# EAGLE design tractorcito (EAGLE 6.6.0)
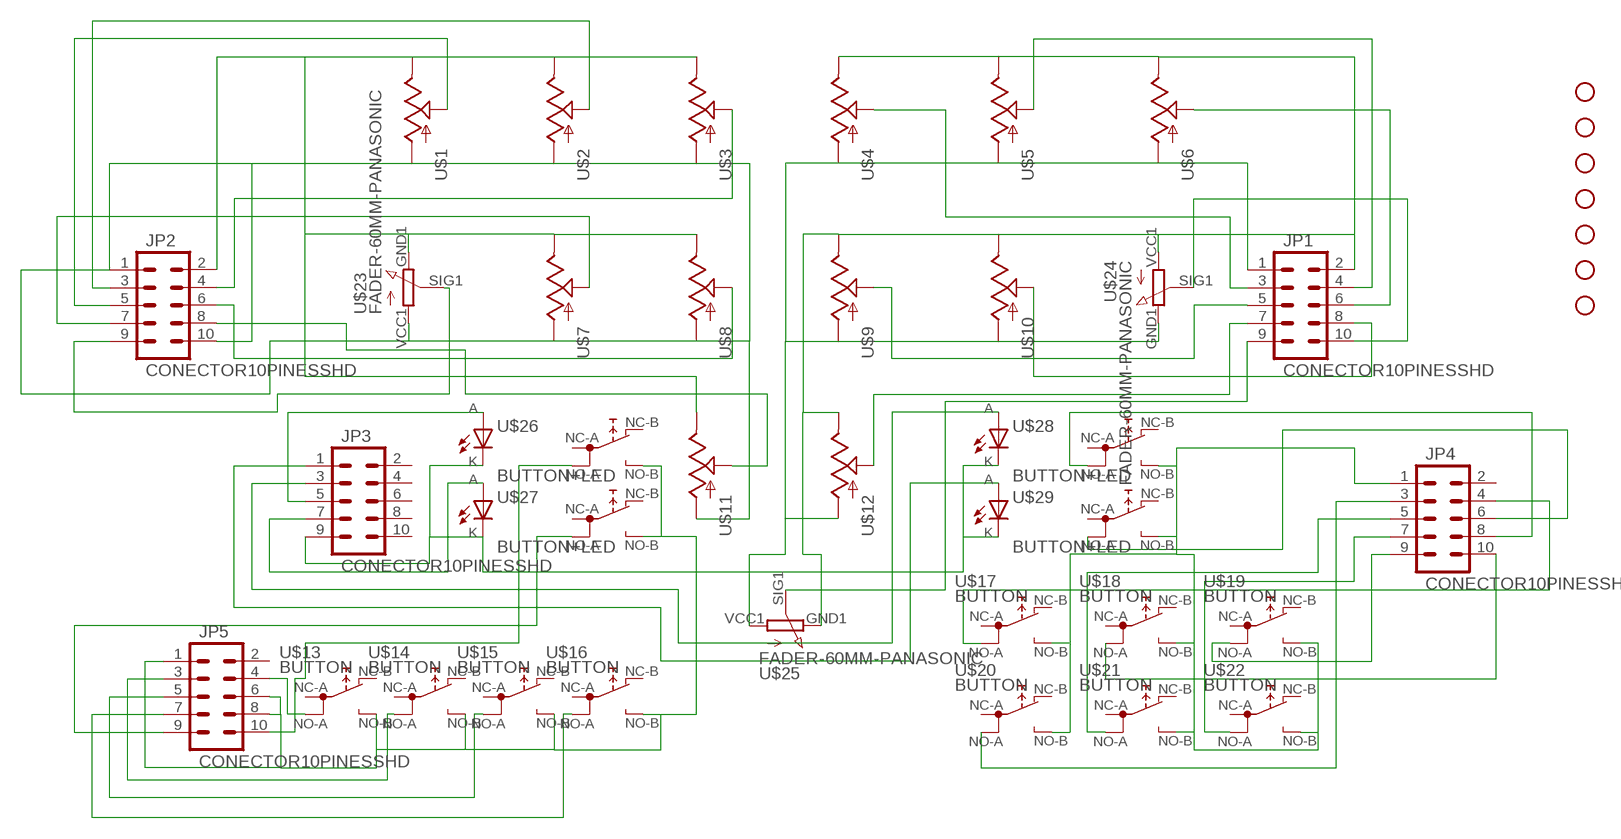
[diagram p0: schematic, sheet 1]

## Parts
JP1  CONECTOR10PINESSHD  [CONECTOR10PINES]
JP2  CONECTOR10PINESSHD  [CONECTOR10PINES]
JP3  CONECTOR10PINESSHD  [CONECTOR10PINES]
JP4  CONECTOR10PINESSHD  [CONECTOR10PINES]
JP5  CONECTOR10PINESSHD  [CONECTOR10PINES]
STANDOFF1  STAND-OFF  [STAND-OFF]
STANDOFF2  STAND-OFF  [STAND-OFF]
STANDOFF3  STAND-OFF  [STAND-OFF]
STANDOFF4  STAND-OFF  [STAND-OFF]
STANDOFF5  STAND-OFF  [STAND-OFF]
STANDOFF6  STAND-OFF  [STAND-OFF]
STANDOFF7  STAND-OFF  [STAND-OFF]
U$1  POT  [ALPS_POT]
U$2  POT  [ALPS_POT]
U$3  POT  [ALPS_POT]
U$4  POT  [ALPS_POT]
U$5  POT  [ALPS_POT]
U$6  POT  [ALPS_POT]
U$7  POT  [ALPS_POT]
U$8  POT  [ALPS_POT]
U$9  POT  [ALPS_POT]
U$10  POT  [ALPS_POT]
U$11  POT  [ALPS_POT]
U$12  POT  [ALPS_POT]
U$13  BUTTON  [BUTTON]
U$14  BUTTON  [BUTTON]
U$15  BUTTON  [BUTTON]
U$16  BUTTON  [BUTTON]
U$17  BUTTON  [BUTTON]
U$18  BUTTON  [BUTTON]
U$19  BUTTON  [BUTTON]
U$20  BUTTON  [BUTTON]
U$21  BUTTON  [BUTTON]
U$22  BUTTON  [BUTTON]
U$23  FADER-60MM-PANASONIC  [FADER-60MM-PANASONIC]
U$24  FADER-60MM-PANASONIC  [FADER-60MM-PANASONIC]
U$25  FADER-60MM-PANASONIC  [FADER-60MM-PANASONIC]
U$26  BUTTON+LED  [BUT+LED]
U$27  BUTTON+LED  [BUT+LED]
U$28  BUTTON+LED  [BUT+LED]
U$29  BUTTON+LED  [BUT+LED]

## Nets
N$1: JP2.2 U$1.P$1(E) U$2.P$1(E) U$3.P$1(E) U$7.P$1(E) U$8.P$1(E) U$11.P$1(E) U$23.GND1
N$2: JP3.9 U$26.K(C) U$27.K(C) U$28.K(C) U$29.K(C)
N$3: JP2.3 U$2.P$2(S)
N$4: JP2.5 U$1.P$2(S)
N$5: JP1.10 U$24.SIG1
N$6: JP2.7 U$7.P$2(S)
N$7: JP2.4 U$3.P$2(S)
N$8: JP2.6 U$8.P$2(S)
N$10: JP1.2 U$4.P$1(E) U$5.P$1(E) U$6.P$1(E) U$9.P$1(E) U$10.P$1(E) U$12.P$1(E) U$24.VCC1 U$25.GND1
N$11: JP1.4 U$5.P$2(S)
N$12: JP1.1 U$4.P$3(A) U$5.P$3(A) U$6.P$3(A) U$9.P$3(A) U$10.P$3(A) U$12.P$3(A) U$24.GND1 U$25.VCC1
N$13: JP1.6 U$6.P$2(S)
N$15: JP1.8 U$10.P$2(S)
N$16: JP1.3 U$4.P$2(S)
N$17: JP1.5 U$9.P$2(S)
N$18: JP1.7 U$12.P$2(S)
N$19: JP4.10 U$18.P$5(1B)
N$20: JP1.9 U$25.SIG1
N$21: JP3.5 U$26.A
N$22: JP3.7 U$27.A
N$23: JP2.9 U$23.SIG1
N$24: JP3.3 U$28.A
N$25: JP3.1 U$29.A
N$26: JP2.1 JP2.10 U$1.P$3(A) U$2.P$3(A) U$3.P$3(A) U$7.P$3(A) U$8.P$3(A) U$11.P$3(A) U$23.VCC1
N$27: JP5.4 U$13.P$5(1B)
N$28: JP5.3 U$14.P$5(1B)
N$29: JP5.5 U$15.P$5(1B)
N$30: JP5.7 U$16.P$5(1B)
N$31: JP5.9 U$27.P$5(1B)
N$32: JP5.10 U$26.P$5(1B)
N$33: JP4.1 U$17.P$6(NO) U$18.P$6(NO) U$19.P$6(NO) U$20.P$6(NO) U$21.P$6(NO) U$22.P$6(NO) U$28.P$6(NO) U$29.P$6(NO)
N$34: JP4.9 U$19.P$5(1B)
N$35: JP4.7 U$22.P$5(1B)
N$36: JP4.5 U$21.P$5(1B)
N$37: JP4.3 U$20.P$5(1B)
N$38: JP4.8 U$28.P$5(1B)
N$39: JP4.4 U$17.P$5(1B)
N$40: JP4.6 U$29.P$5(1B)
N$41: JP5.1 JP5.6 JP5.8 U$13.P$6(NO) U$14.P$6(NO) U$15.P$6(NO) U$16.P$6(NO) U$26.P$6(NO) U$27.P$6(NO)
N$42: JP2.8 U$11.P$2(S)
Unconnected: JP3.2 JP3.4 JP3.6 JP3.8 JP3.10 JP4.2 JP5.2 U$13.P$1(1A) U$13.P$2(NC) U$14.P$1(1A) U$14.P$2(NC) U$15.P$1(1A) U$15.P$2(NC) U$16.P$1(1A) U$16.P$2(NC) U$17.P$1(1A) U$17.P$2(NC) U$18.P$1(1A) U$18.P$2(NC) U$19.P$1(1A) U$19.P$2(NC) U$20.P$1(1A) U$20.P$2(NC) U$21.P$1(1A) U$21.P$2(NC) U$22.P$1(1A) U$22.P$2(NC) U$26.P$1(1A) U$26.P$2(NC) U$27.P$1(1A) U$27.P$2(NC) U$28.P$1(1A) U$28.P$2(NC) U$29.P$1(1A) U$29.P$2(NC)

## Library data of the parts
JP1-JP5 = tcmidi:CONECTOR10PINES: Header 5x2 Standard 10-pin dual row 0.1" header. Commonly used with AVR-ISP. Use with Spark Fun Electronics SKU: PRT-00778
STANDOFF1-STANDOFF7 = SparkFun-Electromechanical:STAND-OFF: #4 Stand Off
U$1-U$12 = SparkFun-Electromechanical:POT
U$13-U$22 = tcmidi:BUTTON
U$23-U$25 = tcmidi:FADER-60MM-PANASONIC
U$26-U$29 = tcmidi:BUTTON+LED

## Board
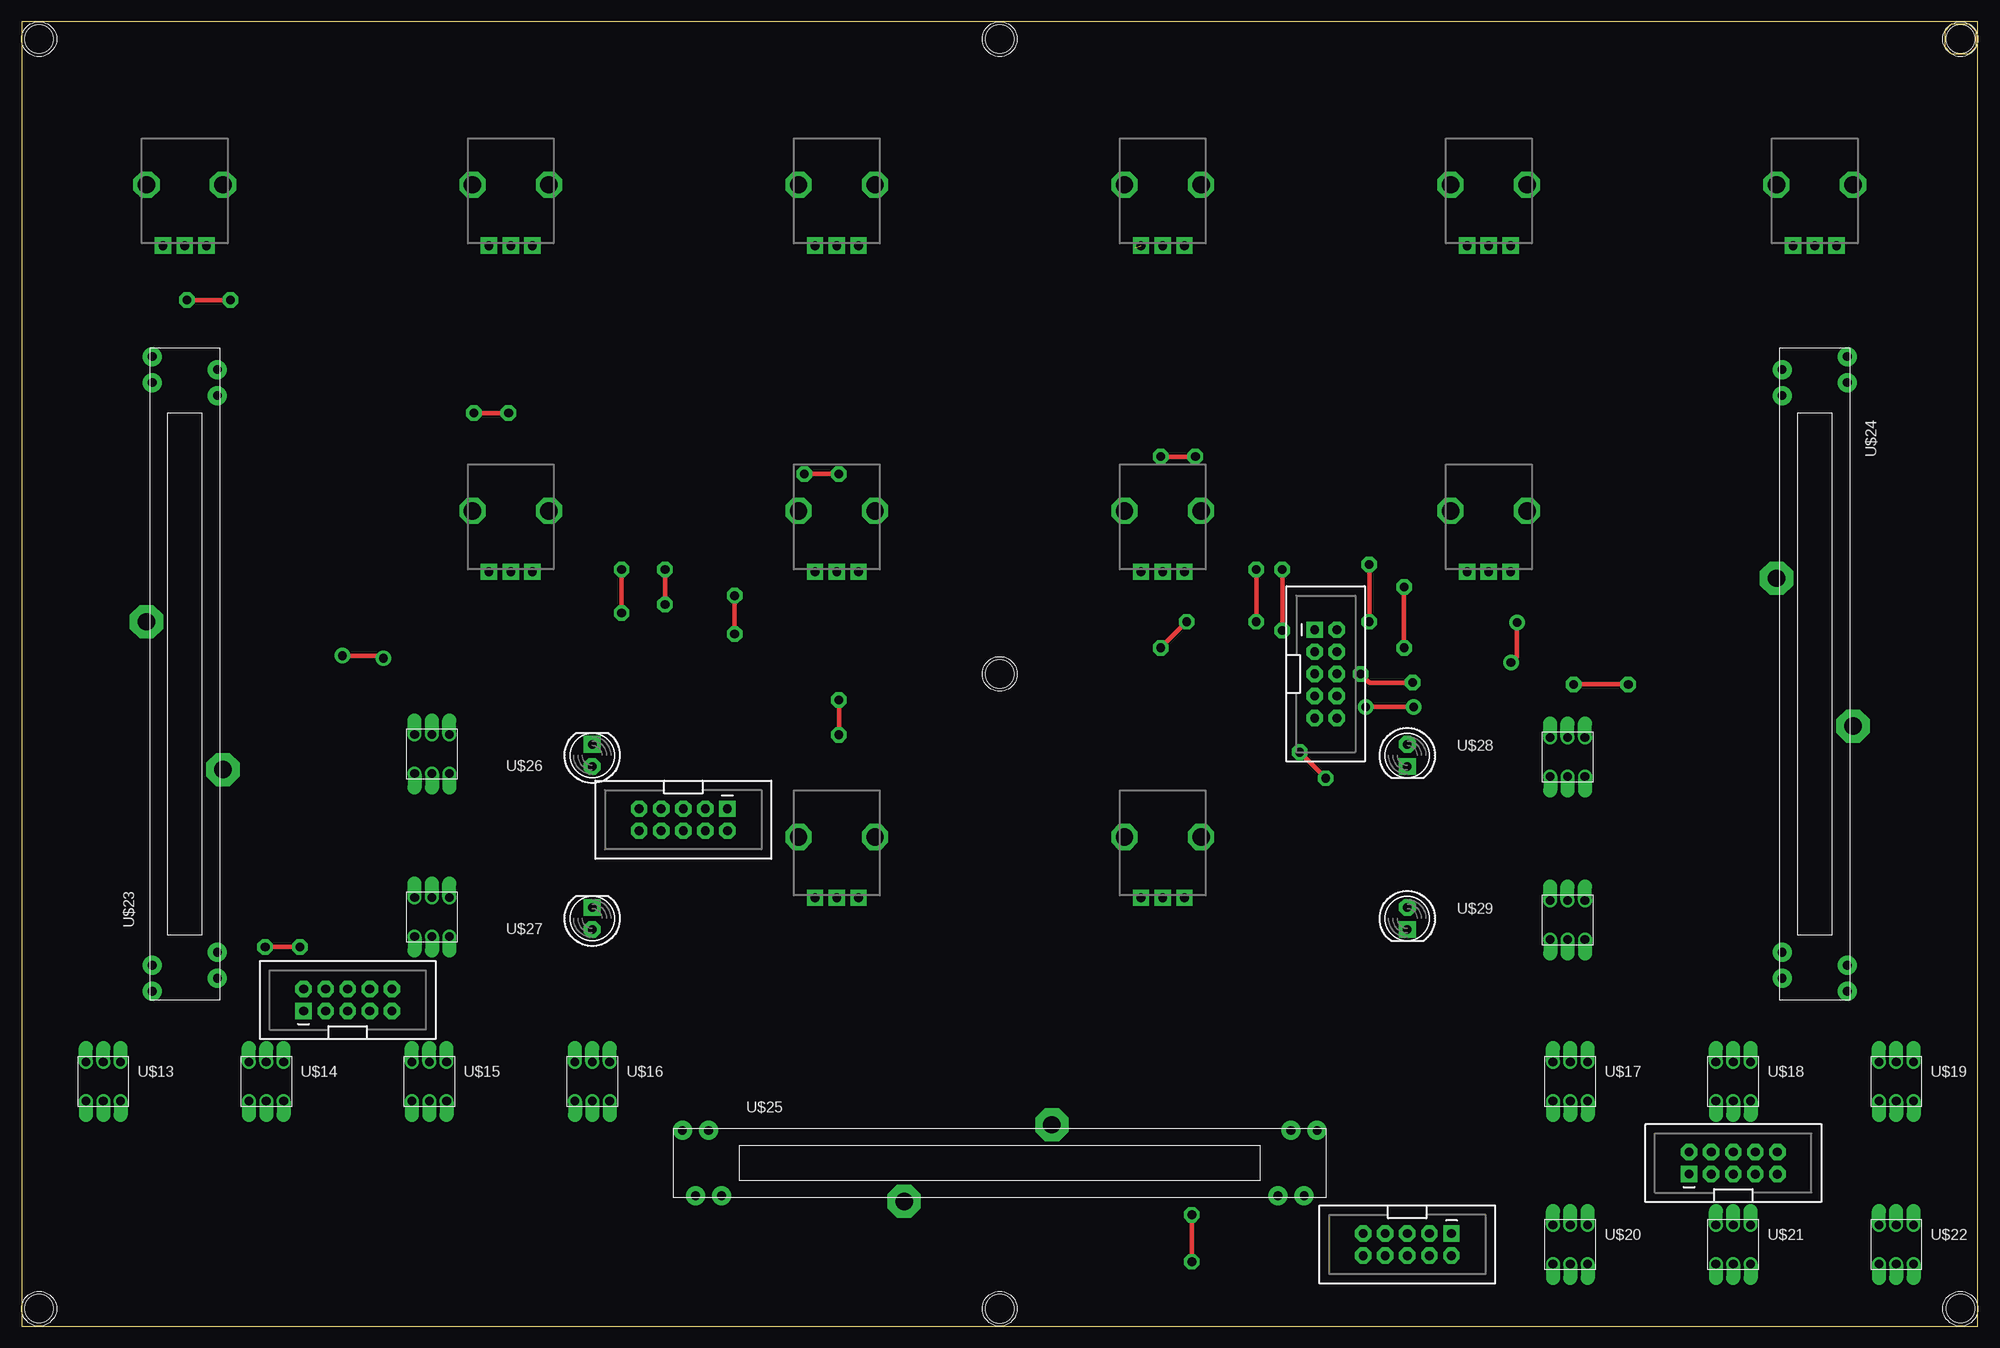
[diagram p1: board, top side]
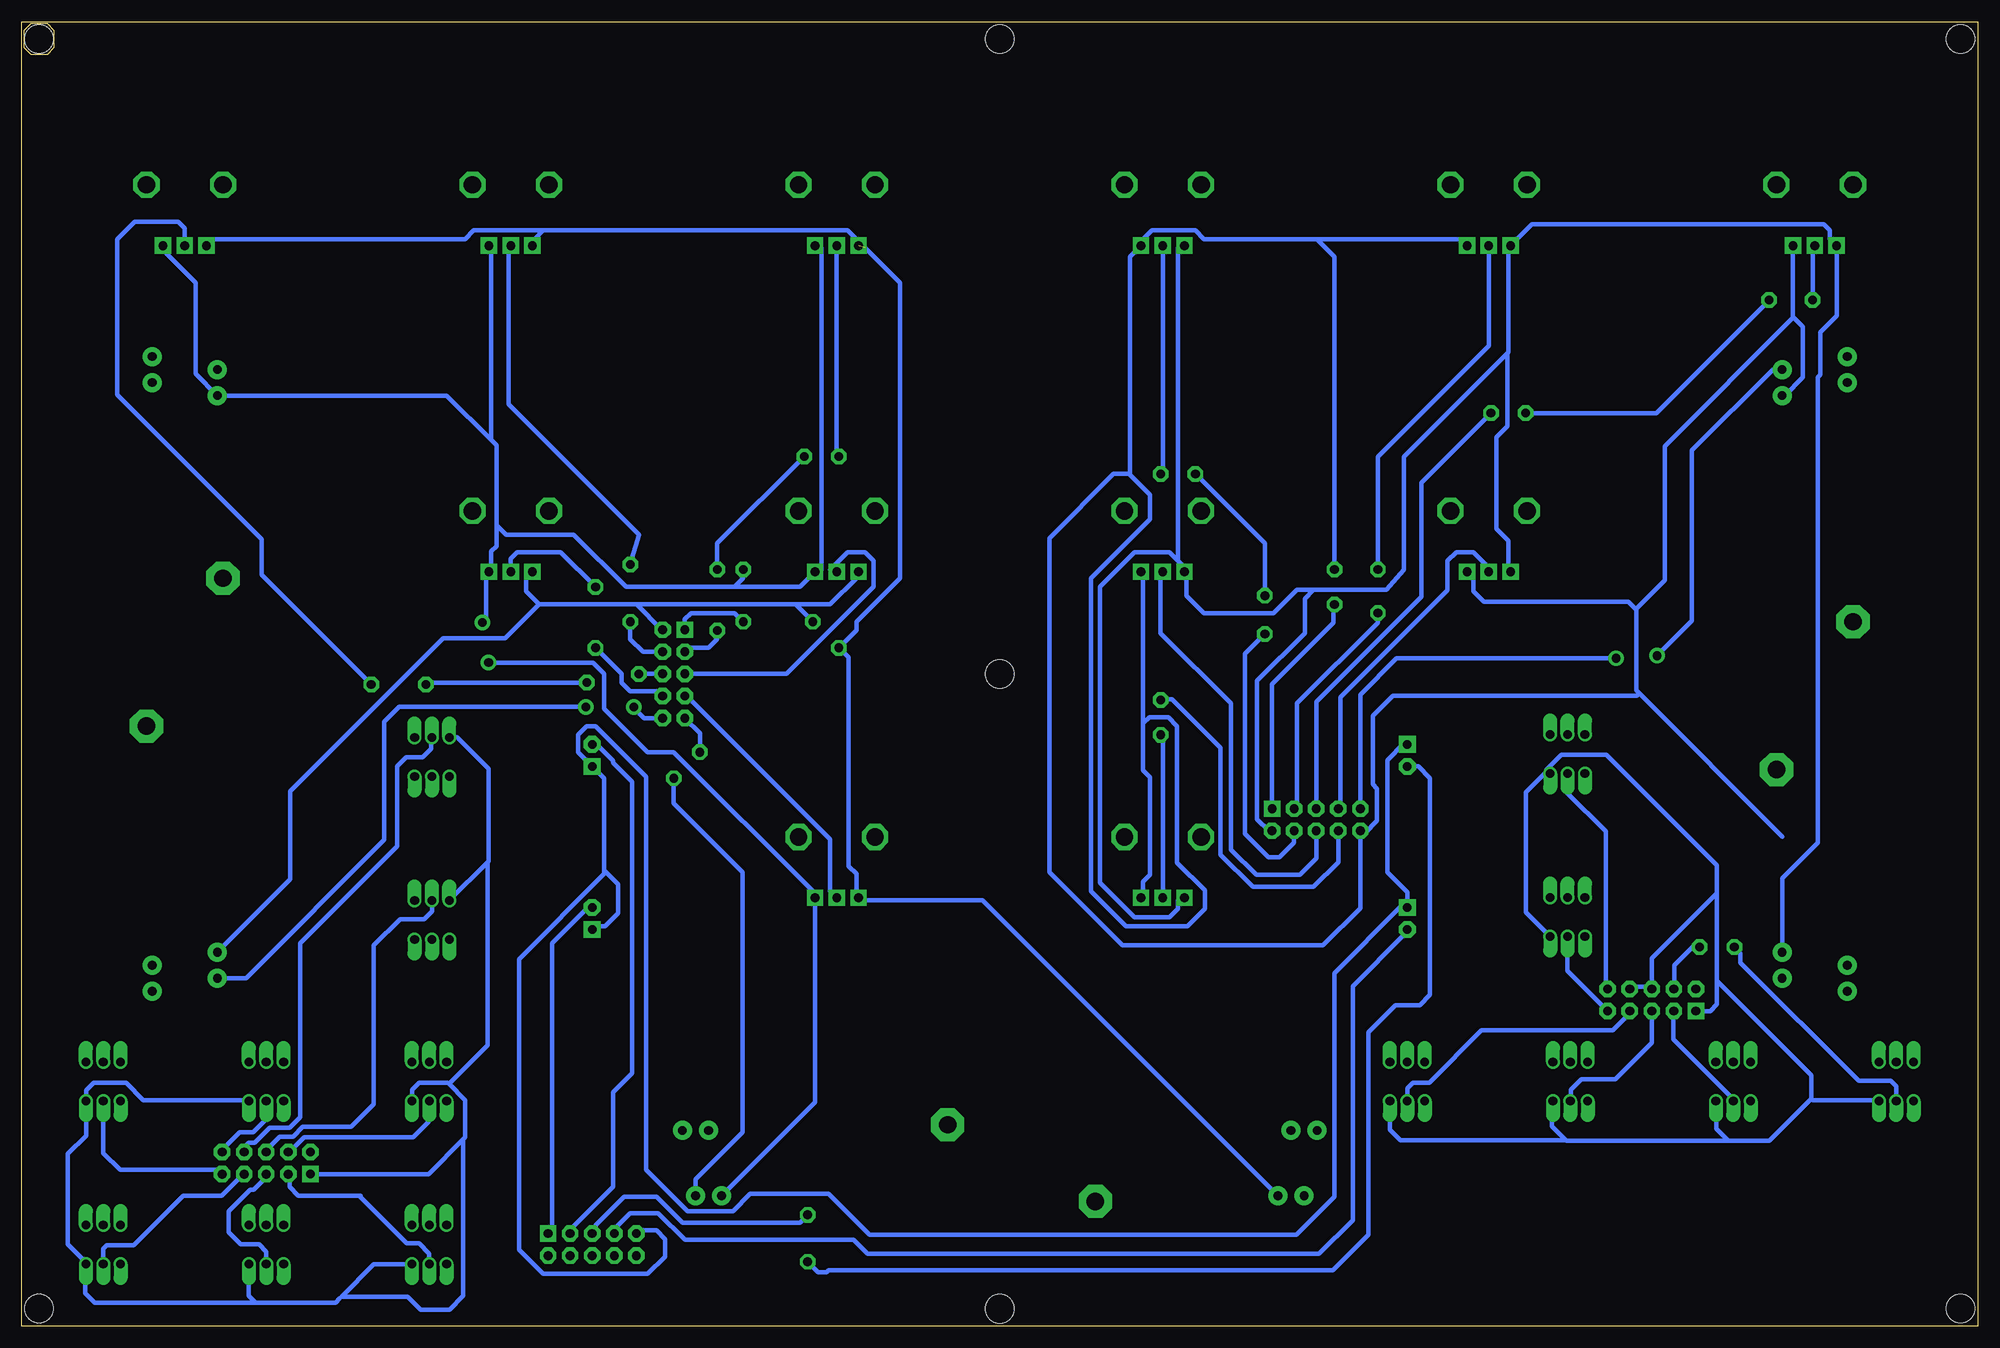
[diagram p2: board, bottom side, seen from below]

Size 225 x 150 mm. Coordinates in mm from the lower left corner, seen from the top.
Outline: 0,0 225,0 225,150 0,150 0,0
Outline: 224.75,147.04 223.97,146.26 222.04,146.26 221.25,147.04 221.25,148.97 222.04,149.76 223.97,149.76 224.75,148.97 224.75,147.04
Copper layers (1*16): Top 0.035mm / dielectric 1.5mm / Bottom 0.035mm
Design rules "tcmidi *": minimum track width 14mil, minimum drill 20mil, track to track 16mil, track to pad 16mil, pad to pad 12mil, via to via 16mil, smd to smd 16mil, copper to edge 16mil, drill to drill 16mil, minimum pad ring 12mil, minimum via ring 10mil, stop-mask expansion 4mil, vias tented up to drill 20mil, thermal gap 10mil

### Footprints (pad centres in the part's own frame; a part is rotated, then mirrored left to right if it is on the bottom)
CONECTOR10PINES = drill 1 pad 1.88 square: 1 -1.27,5.08 | drill 1.016 pad 1.88 octagon: 2 1.27,5.08; 3 -1.27,2.54; 4 1.27,2.54; 5 -1.27,0; 6 1.27,0; 7 -1.27,-2.54; 8 1.27,-2.54; 9 -1.27,-5.08; 10 1.27,-5.08
STAND-OFF = hole 3.302: 0,0
ALPS_POT = drill 1 pad 1.88 square: P$1 7,-2.5; P$2 7,0; P$3 7,2.5 | drill 2 octagon: P$4 0,-4.4; P$5 0,4.4
BUTTON = drill 1 pad 1.5 offset: P$1 -2,2.25; P$2 0,2.25; P$3 2,2.25; P$4 -2,-2.25; P$5 0,-2.25; P$6 2,-2.25
FADER-60MM-PANASONIC = drill 1 pad 2.184: GND1 -32,-3.75; GND2 -33.5,3.75; GND11 -35,-3.75; GND22 -36.5,3.75; SIG1 35,-3.75; SIG2 36.5,3.75; VCC1 32,-3.75; VCC2 33.5,3.75 | drill 2 pad 3.81 octagon: P$9 -11,-4.4; P$10 6,4.4
BUT+LED = drill 1 pad 1.93 octagon: A -9.375,1.27 | drill 1 pad 1.93 square: K -9.375,-1.27 | drill 1 pad 1.5 offset: P$1 11.06,-2.42; P$2 9.06,-2.42; P$3 7.06,-2.42; P$4 11.06,2.08; P$5 9.06,2.08; P$6 7.06,2.08

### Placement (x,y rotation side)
JP1  150,75 0 top
JP2  76.1,58.23 270 top
JP3  159.38,9.38 270 top
JP4  196.88,18.75 90 top
JP5  37.5,37.5 90 top
STANDOFF1  2,2 0 top
STANDOFF2  112.5,1.99 0 top
STANDOFF3  223,2 0 top
STANDOFF4  2,148 0 top
STANDOFF5  112.5,148 0 top
STANDOFF6  223,148 0 top
STANDOFF7  112.5,75 0 top
U$1  18.75,131.25 270 top
U$2  56.25,131.25 270 top
U$3  93.75,131.25 270 top
U$4  131.25,131.25 270 top
U$5  168.75,131.25 270 top
U$6  206.25,131.25 270 top
U$7  56.25,93.75 270 top
U$8  93.75,93.75 270 top
U$9  131.25,93.75 270 top
U$10  168.75,93.75 270 top
U$11  93.75,56.25 270 top
U$12  131.25,56.25 270 top
U$13  9.38,28.12 0 top
U$14  28.12,28.12 0 top
U$15  46.88,28.12 0 top
U$16  65.62,28.12 0 top
U$17  178.12,28.12 0 top
U$18  196.88,28.12 0 top
U$19  215.62,28.12 0 top
U$20  178.12,9.38 0 top
U$21  196.88,9.38 0 top
U$22  215.62,9.38 0 top
U$23  18.75,75 90 top
U$24  206.25,75 270 top
U$25  112.5,18.75 0 top
U$26  56.25,65.62 180 top
U$27  56.25,46.88 180 top
U$28  168.75,65.62 0 top
U$29  168.75,46.88 0 top

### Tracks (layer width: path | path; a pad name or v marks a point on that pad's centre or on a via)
N$1
  Bottom 0.508: U$7.P$1 54,87 54,90.3 55.4,91.7 55.4,102.2 54.1,103.5 54.1,111.9 | 92,88 91,87 U$8.P$1 91,86 91,84 89,82 81.03,82 78.34,84.65 76.4,84.66 | 92,88 93,89 97,89 101,85 101,51 97,47 93,47 92,48 92,49 U$11.P$1 | 92,88 92,124 U$3.P$1 | 54.1,111.9 66,100 66,87 68.03,84.68 76.4,84.66 | 54.1,111.9 54,112 54,124 U$2.P$1 51.3,126.7 17.7,126.7 17,126 17,125 U$1.P$1 16.2,124.2 16.2,116.2 18.1,114.3 18.1,109.4 18.4,109.1 18.4,55.6 22.5,51.5 U$23.GND1 | JP2.2 81.56,56.95 82.9,58.3 82.9,74.2 77.4,79.7 77.4,83.66 76.4,84.66
N$2
  Bottom 0.508: U$26.K 66,67 67.9,65.1 67.9,52.2 65.6,49.9 65.6,48.17 U$27.K 66.45,48.15 74,40.6 74,14.9 78.4,10.5 127.5,10.5 132.2,15.2 141.2,15.2 143.2,13.2 148.4,13.2 153.2,18 153.2,63.2 159,69 160,69 161,68 161,66 160,65 U$28.K 159,64 158,63 158,52.4 | 158,52.4 158,52 167.8,42.2 167.8,8.8 165,6 153,6 151,8 151,10 152,11 153.94,11 JP3.9 | U$29.K 159,46 157.9,46 156.4,47.5 156.4,50.8 158,52.4
N$3  (via drill 1 pad 1.78)
  Top 0.508: v69,87 v69,82
  Bottom 0.508: U$2.P$2 56.25,112.75 69,100 v69,87 | v69,82 69,80.9 78.3,71.6 78.3,59.84 JP2.3
N$4  (via drill 1 pad 1.78)
  Top 0.508: v56,105 v52,105 | v24,118 v19,118
  Bottom 0.508: v56,105 64,97 64,83.9 76.1,71.8 JP2.5 | v52,105 37,105 v24,118 | v19,118 19,124 U$1.P$2
N$5  (via drill 1 pad 1.78)
  Top 0.508: v160.1,71.2 v154.6,71.2
  Bottom 0.508: U$24.SIG1 199.2,40 183.3,55.9 183.3,69.5 181.6,71.2 v160.1,71.2 | v154.6,71.2 154.6,71.1 153.4,69.9 151.29,69.9 JP1.10
N$6
  Bottom 0.508: U$7.P$2 56,87 58,89 60,89 61,88 61,84.6 73.3,72.3 73.3,59.76 JP2.7
N$7  (via drill 1 pad 1.78)
  Top 0.508: v94,98 v90,98 | v82,84 v82,79.6
  Bottom 0.508: U$3.P$2 93.75,98.25 v94,98 | v82,84 82,90 v90,98 | JP2.4 78.64,55.56 80.3,53.9 81.6,53.9 84.3,56.6 84.3,77.3 v82,79.6
N$8
  Bottom 0.508: JP2.6 76.1,53.8 78,51.9 83,51.9 85.9,54.8 85.9,71.6 94,79.7 94,86.5 U$8.P$2
N$10  (via drill 1 pad 1.78)  (1 unrouted)
  Top 0.508: v131,78 v134,81
  Bottom 0.508: U$10.P$1 167,86 167,84.5 165.5,83 | 154.3,83 136,83 | U$9.P$1 129,86 132,83 136,83 | 128,124 124,120 124,86 129,81 129,80 v131,78 129.9,76.9 129.9,52.9 129,52 129,50 U$12.P$1 128,49 114.5,49 U$25.GND1 | v134,81 136,83 | 165,126 130,126 129,125 U$4.P$1 | 165,126 166,125 U$5.P$1 | 165,126 173,126 174,125 203,125 U$6.P$1 | JP1.2 151.38,80.08 154.3,83 | 165.5,83 154.3,83 | 165.5,83 169.4,79.1 176.5,79.1 194.1,61.5 194.1,51.4 U$24.VCC1
N$11  (via drill 1 pad 1.78)
  Top 0.508: v155,81 v155,87.6
  Bottom 0.508: JP1.4 153.54,77.54 155,79 v155,81 | v155,87.6 154,91 169,106 169,124 U$5.P$2
N$12  (via drill 1 pad 1.78)
  Top 0.508: v142,81 v142,87 | v172,80.9 172,77 v171.3,76.3
  Bottom 0.508: U$4.P$3 133,124 133,87 U$9.P$3 135.5,85 143,85 | U$6.P$3 209,124 205,120 205,109.5 U$24.GND1 176.1,107 171,101.9 | 171,101.9 171,124 U$5.P$3 | 143,85 155.5,85 161.5,91 169.3,91 170.4,92.1 | JP1.1 148.73,81.27 148,82 143,82 v142,81 | v142,87 142,86 143,85 | 170.4,92.1 170.4,89.7 171,89.1 171,87 U$10.P$3 171.6,86.4 171.6,81.3 v172,80.9 | 170.4,92.1 170.4,101.3 171,101.9 | U$25.VCC1 133.75,25.75 U$12.P$3 134,50 150,66 153,66 158,71 158,75 159.3,76.3 v171.3,76.3
N$13  (via drill 1 pad 1.78)
  Top 0.508: v184.8,73.8 v178.5,73.8 | v160,74 155,74 v154,75
  Bottom 0.508: U$6.P$2 206.25,126.25 207,127 212,127 214,125 214,107.1 197.4,90.5 197.4,86.4 v184.8,73.8 | v178.5,73.8 178,74 v160,74 | v154,75 JP1.6
N$15  (via drill 1 pad 1.78)
  Top 0.508: v159,85 v159,78
  Bottom 0.508: U$10.P$2 168.75,88.25 168,89 163,89 v159,85 | v159,78 156,75 156,74 155,73 151.81,73 JP1.8
N$16  (via drill 1 pad 1.78)
  Top 0.508: v131,100 v135,100 | v145,87 v145,80
  Bottom 0.508: U$4.P$2 131.25,100.25 v131,100 | v135,100 145,90 v145,87 | v145,80 145,79 146,78 148.27,78 JP1.3
N$17
  Bottom 0.508: JP1.5 137,75 127,85 127,88 128,89 130,89 132,87 U$9.P$2
N$18
  Bottom 0.508: U$12.P$2 132,50 132,56 148,72 JP1.7
N$19
  Bottom 0.508: JP4.10 202,20 202,20.2 199.9,22.3 198.4,22.3 197,23.7 197,25.75 U$18.P$5
N$20  (via drill 1 pad 1.78)
  Top 0.508: v150,63 v147,66
  Bottom 0.508: v150,63 150,60.1 142.1,52.2 142.1,22.3 147.5,16.9 U$25.SIG1 | v147,66 147,68.19 JP1.9
N$21  (via drill 1 pad 1.78)
  Top 0.508: v134.6,7.4 v134.6,12.8
  Bottom 0.508: U$26.A 64.36,64.36 63,63 63,38.1 64.2,36.9 67,36.9 70.1,33.8 70.1,10.5 74.2,6.4 132.2,6.4 132.4,6.2 133.4,6.2 v134.6,7.4 | JP3.5 159,11.02 159,11.6 155.7,14.9 152,14.9 149,11.9 135.5,11.9 v134.6,12.8
N$22
  Bottom 0.508: U$27.A 66,45 71.9,39.1 71.9,12.2 75.8,8.3 127.7,8.3 129.3,9.9 148.7,9.9 151.8,13 155,13 157,11 JP3.7
N$23  (via drill 1 pad 1.78)
  Top 0.508: v36.9,77.1 41.3,77.1 v41.6,76.8
  Bottom 0.508: v36.9,77.1 32.9,81.1 32.9,100.7 23.6,110 U$23.SIG1 | v41.6,76.8 66.85,76.8 71.02,72.63 JP2.9
N$24
  Bottom 0.508: U$28.A 159,67 157,65 157,64.8 154.8,62.6 154.8,29.1 157,26.9 157,16 162,11 JP3.3
N$25
  Bottom 0.508: U$29.A 160,48 164,44 164,11 JP3.1
N$26  (via drill 1 pad 1.78)
  Top 0.508: v74,83 v74,87
  Bottom 0.508: U$7.P$3 58,86 58,84.5 56.8,83.3 40.2,83.3 39.35,82.45 | 76,125 89,125 90,126 95,126 96,125 U$3.P$3 97.5,123 97.5,98 | 76,125 59,125 U$2.P$3 | 96,69.3 96,86 U$8.P$3 | U$11.P$3 96,50 96,51.1 95.2,51.9 95.2,63.1 96,63.9 96,69.3 | 96,69.3 95.3,70 93.1,70 92.1,69 92.1,53.3 88.9,50.1 88.9,48 90.9,46 98,46 102,50 102,86 95.2,92.8 95.2,95.6 97.5,97.9 97.5,98 | v74,87 74,123 76,125 | U$1.P$3 21.25,116.1 | 21.25,116.1 21.25,115.95 36,101.2 36,85.8 39.35,82.45 | 22.5,56.3 38.95,72.75 | 38.95,72.75 39.3,73.1 39.3,82.4 39.35,82.45 | 97.5,98 99.4,98 106.8,90.6 106.8,52.2 98.4,43.8 75.3,43.8 71.02,48.08 JP2.10 70.77,56.7 70.5,56.7 69.1,58.1 69.1,61.8 69.6,62.3 69.6,70.2 67.3,72.5 39.2,72.5 38.95,72.75 | JP2.1 81.18,73.82 74.1,80.9 74.1,82.9 v74,83 | U$23.VCC1 22.2,107 20.1,109.1 20.1,114.95 21.25,116.1
N$27  (via drill 1 pad 1.78)
  Top 0.508: v28,43.6 v32,43.6
  Bottom 0.508: U$13.P$5 9.38,27.57 10,28.2 13.7,28.2 27.3,41.8 27.3,42.9 v28,43.6 | v32,43.6 32.8,43.6 34.9,41.5 34.9,38.83 JP5.4
N$28
  Bottom 0.508: U$14.P$5 28,26 35,33 35,36 JP5.3
N$29
  Bottom 0.508: JP5.5 37.5,32.6 41.7,28.4 45.6,28.4 46.8,27.2 46.8,25.95 U$15.P$5
N$30
  Bottom 0.508: JP5.7 40,36 42,34 57.1,34 63.1,28 65,28 65.62,27.38 U$16.P$5
N$31
  Bottom 0.508: U$27.P$5 47.19,40.84 JP5.9
N$32
  Bottom 0.508: 43,39 JP5.10 42.8,38.99 42.8,56.9 47.19,61.29 U$26.P$5
N$33
  Bottom 0.508: U$18.P$6 199,26 211,26 213,28 216.7,28 217.6,27.1 217.6,25.9 U$19.P$6 217.6,25.85 217.6,21.9 219.7,19.8 219.7,9.4 217.62,7.33 U$22.P$6 217.7,7.05 217.7,3.8 216.6,2.7 198.1,2.7 | 180,7 U$20.P$6 180.15,7.1 184.5,7.1 188.2,3.4 | 199,7 U$21.P$6 198.9,7.1 198.9,3.5 198.1,2.7 | 175.85,27.85 174,26 174,21.7 174.2,21.5 | 175.85,27.85 176,28 179.3,28 180.1,27.2 180.1,25.9 U$17.P$6 | JP4.1 178.22,17.48 174.2,21.5 | U$28.P$6 174.91,67.7 171.3,64.1 171.3,53.47 171.43,53.34 | 171.43,53.34 U$29.P$6 | 171.43,53.34 171.43,32.27 175.85,27.85 | 174.2,21.5 174.2,3.5 175.8,1.9 179.1,1.9 180.6,3.4 188.2,3.4 | 198.1,2.7 188.9,2.7 188.4,3.2 188.2,3.4
N$34
  Bottom 0.508: JP4.9 202,18 213.7,18 215.6,19.9 215.6,25.85 U$19.P$5
N$35
  Bottom 0.508: JP4.7 200,17 202,15 206.4,15 212.1,9.3 215.2,9.3 215.62,8.88 U$22.P$5
N$36
  Bottom 0.508: JP4.5 197,17 198.3,15.7 198.7,15.7 201.2,13.2 201.2,10.8 199.8,9.4 197.7,9.4 196.88,8.57 U$21.P$5
N$37
  Bottom 0.508: 186.2,15 193.2,15 194.2,16 194.2,17.34 JP4.3 | 186.2,15 186,15 | U$20.P$5 178.12,8.32 179.3,9.5 180.7,9.5 186.2,15
N$38
  Bottom 0.508: U$28.P$5 177.9,67.61 177.9,66.4 178.9,65.4 180.8,65.4 181.8,64.4 181.8,55.2 193,44 193,24 194.2,22.8 196.5,22.8 198.2,21.1 198.9,21.1 199.41,20.59 JP4.8
N$39
  Bottom 0.508: U$17.P$5 178.2,25.8 178.2,23.5 179.5,22.2 179.7,22 180,21.7 192.5,21.7 194.18,20.02 JP4.4
N$40
  Bottom 0.508: JP4.6 197,20 197,20.1 195.3,21.8 193.8,21.8 192.7,22.9 187.1,22.9 184.5,25.5 184.5,43.8 181.5,46.8 178.7,46.8 177.81,47.69 U$29.P$5
N$41
  Bottom 0.508: JP5.8 40,39 38,39 JP5.6 37.5,42.3 30,49.8 | 19.15,26.15 19,26 12,26 U$13.P$6 | 30,49.8 30,53 42.7,65.7 47.9,65.7 49.6,64 49.6,63.65 49.7,63.55 | 30,49.8 30,39.7 | 30,39.7 30,37 30.77,36.23 JP5.1 | U$15.P$6 49,26 49,23 47.4,21.4 | U$26.P$6 49.7,63.55 | 49.7,63.55 49.85,63.55 52,61.4 52,47.6 U$27.P$6 | 19.15,26.15 19.15,28.85 30,39.7 | 19.15,26.15 24,21.3 28.7,21.3 | 28.7,21.3 30.1,22.7 30.1,25.85 U$14.P$6 | 28.7,21.3 47.3,21.3 47.4,21.4 | 47.4,21.4 66.4,21.4 67.6,22.6 67.6,25.85 U$16.P$6
N$42  (via drill 1 pad 1.78)
  Top 0.508: v94,68 v94,72
  Bottom 0.508: U$11.P$2 93.75,67.75 v94,68 | v94,72 93.9,72.1 92.7,72.1 87.1,66.5 87.1,54.2 83.4,50.5 76.4,50.5 73.56,53.34 JP2.8

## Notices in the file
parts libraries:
SparkFun-Electromechanical: Licensing: CC v3.0 Share-Alike You are welcome to use this library for commercial purposes.
